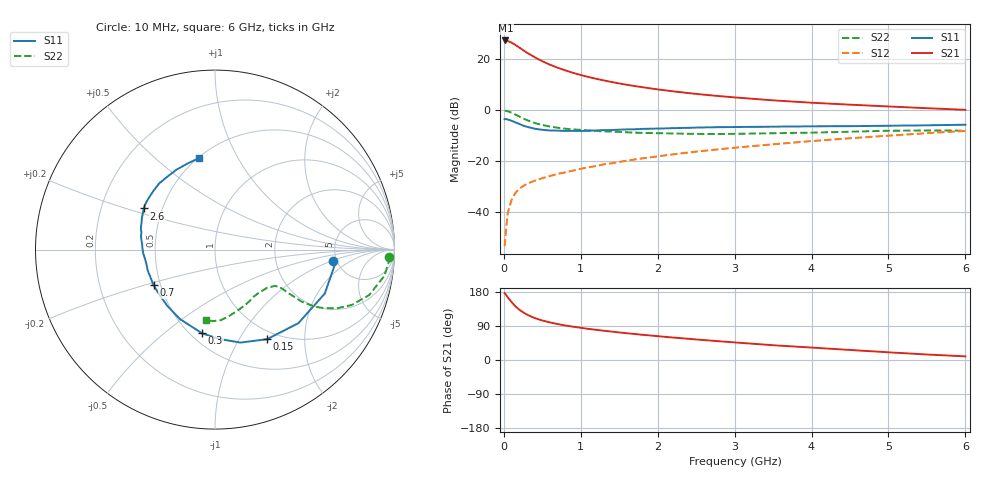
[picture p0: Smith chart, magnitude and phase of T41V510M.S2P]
! Infineon Technologies  Discrete & RF Semiconductors
! BFR182T
! Si NPN RF Bipolar Junction Transistor in SC75
! VCE = 1.5 V  IC = 10 mA
! Common Emitter S-Parameters:  October  1999
# GHz  S  MA  R  50
!  f  S11  S21  S12  S22
! GHz  MAG  ANG  MAG  ANG  MAG  ANG  MAG  ANG
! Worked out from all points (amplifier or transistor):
!   36 points, 10 MHz to 6 GHz, reference 50 ohm
!   highest |S21| = 27.5 dB at 20 MHz (marker M1)
!   |S21| within 3 dB of that: start of sweep to 211.7 MHz
!   unconditionally stable (mu >= 1): 874.3 MHz to 3.888 GHz
!   at 250 MHz: K = 0.47, MSG = 26.8 dB, |S12| = -29.9 dB
!   at 1.4 GHz: K = 1.11, MAG = 14.0 dB, |S12| = -20.9 dB
!   at 6 GHz: K = 0.86, MSG = 4.2 dB, |S12| = -8.2 dB
!   lowest NFmin = 1.50 dB at 450 MHz
!   S11 on the Smith chart (normalised r, x): 10 MHz: 4.66, -1.05; 150 MHz: 0.89, -1.33; 300 MHz: 0.57, -0.68; 700 MHz: 0.46, -0.22; 2.6 GHz: 0.39, +0.23; 6 GHz: 0.51, +0.71
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0.01  0.6616 -5.5  23.57 176.3  0.0021 79.8  0.9686 -2.5
0.02  0.6724 -7.4  23.66 174.4  0.0032 89.0  0.9733 -3.5
0.05  0.659 -21.8  23.12 165.7  0.0093 84.3  0.9549 -8.8
0.1  0.6196 -41.4  21.44 153.0  0.017 73.5  0.896 -16.4
0.15  0.5774 -59.8  19.32 141.8  0.0234 66.5  0.8211 -22.1
0.2  0.5371 -74.7  17.23 132.9  0.0284 62.7  0.7524 -25.8
0.25  0.4986 -87.2  15.29 125.8  0.032 60.0  0.688 -28.3
0.3  0.472 -98.8  13.62 119.9  0.0355 58.6  0.6387 -29.8
0.4  0.4331 -117.0  11.08 110.7  0.0408 56.2  0.5599 -31.0
0.5  0.4109 -130.2  9.231 104.3  0.0459 56.8  0.5115 -30.8
0.6  0.399 -140.8  7.867 99.1  0.0506 57.6  0.4771 -30.7
0.7  0.3959 -149.8  6.868 94.8  0.0558 58.8  0.4511 -30.4
0.9  0.3926 -163.0  5.444 87.9  0.0647 61.5  0.4182 -30.2
1.1  0.3946 -173.5  4.517 82.0  0.075 62.9  0.3994 -30.8
1.3  0.4047 178.7  3.866 77.2  0.086 63.9  0.3835 -32.1
1.6  0.4198 169.3  3.168 70.6  0.1015 65.3  0.3674 -34.4
2.2  0.4432 156.8  2.356 59.3  0.1352 65.9  0.3485 -41.8
2.6  0.4586 150.0  2.024 52.6  0.1587 65.6  0.3409 -47.4
3.5  0.4738 136.5  1.564 39.0  0.2133 63.0  0.3519 -61.3
4.5  0.485 123.6  1.286 26.5  0.2803 58.3  0.3769 -77.4
5.5  0.5042 107.2  1.096 14.5  0.3531 52.4  0.3983 -91.3
6  0.5183 99.6  1.019 9.6  0.3912 48.4  0.3967 -97.1
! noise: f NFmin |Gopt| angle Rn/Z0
0.45  1.5  0.26  43  0.28
0.9  1.6  0.24  87  0.22
1.8  2.1  0.2  170  0.2
